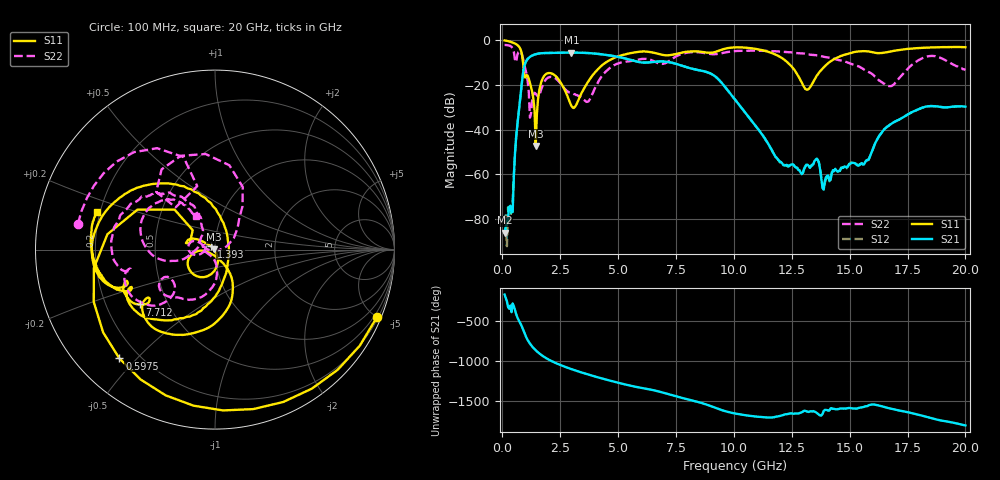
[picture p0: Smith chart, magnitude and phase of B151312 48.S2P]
!  2-Port S-parameters saved by WinCal
! VAR MeasName=S-Parameters (CALIBRATED_DATA) read from VNA (N5244A)
! VAR MeasDate=12/8/2015 5:47:35 PM
! VAR NAME=B151312 48
! VAR FILENAME=B151312 48.S2P
! VAR DATE=12/8/2015 5:47:35 PM
! VAR PHYS_PORTS=1,2
# Hz S DB R 50
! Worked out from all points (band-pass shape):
!   401 points, 100 MHz to 20 GHz, reference 50 ohm
!   highest |S21| = -5.62 dB at 2.986 GHz (marker M1); lowest = -86.1 dB at 100 MHz (marker M2)
!   |S21| within 3 dB of the highest: 1.086 GHz to 5.449 GHz (4.364 GHz wide, 134 % of centre)
!   lowest |S11| = -47.4 dB at 1.443 GHz (marker M3), VSWR 1.01, Z = 49.6 + j0.101 ohm
!   |S11| at or under -10 dB: 896.1 MHz to 4.474 GHz (3.578 GHz wide, 133 % of centre); 12.32 GHz to 14.12 GHz (1.798 GHz wide, 13.6 % of centre)
!   |S22| runs from -34.7 to -2.2 dB; largest |S21 - S12| = 0.0018
!   S11 on the Smith chart (normalised r, x): 100 MHz: 0.29, -4.99; 597.5 MHz: 0.13, -0.45; 1.393 GHz: 0.96, +0.03; 7.712 GHz: 0.35, -0.29; 20 GHz: 0.19, +0.15
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1e8  -0.20 -22.6  -86.13 -169.8  -81.85 -179.3  -2.19 169.3
3.985e8  -0.94 -87.2  -76.92 -30.0  -74.79 8.1  -3.03 129.7
5.975e8  -1.86 -131.3  -43.45 -52.8  -43.50 -52.8  -9.86 132.9
9.4575e8  -15.67 138.9  -11.90 74.9  -11.90 74.8  -10.89 57.6
1.1945e9  -19.11 149.2  -7.51 -63.9  -7.51 -63.9  -34.69 -15.0
1.3935e9  -31.37 139.9  -6.50 -133.2  -6.51 -133.1  -23.60 158.5
1.44325e9  -47.37 166.3  -6.35 -147.4  -6.34 -147.4  -23.99 156.4
1.692e9  -18.49 -91.7  -5.90 152.7  -5.89 152.6  -21.73 -163.1
1.9905e9  -14.77 -130.6  -5.79 98.4  -5.78 98.4  -16.71 -177.6
2.9855e9  -29.43 -144.0  -5.62 -23.0  -5.62 -23.0  -23.76 177.1
3.43325e9  -23.50 -64.8  -5.70 -65.7  -5.70 -65.6  -25.75 -162.9
4.72675e9  -8.51 -84.3  -7.04 -172.5  -7.02 -172.6  -11.89 -101.8
6.7665e9  -6.26 -144.2  -9.58 56.6  -9.58 56.5  -10.47 -148.8
7.71175e9  -5.73 -143.8  -11.36 -19.6  -11.32 -19.7  -6.39 -139.6
1.005e10  -3.28 -175.8  -26.67 141.8  -26.65 141.5  -4.94 -174.0
1.204e10  -7.86 118.6  -54.51 115.4  -54.99 114.6  -5.23 157.2
1.338325e10  -19.56 -47.9  -55.67 167.1  -56.11 169.4  -6.66 138.1
1.388075e10  -12.20 -87.4  -66.76 173.6  -66.85 175.9  -7.49 132.8
1.55225e10  -4.99 -144.7  -54.98 -142.2  -55.09 -142.8  -12.52 116.5
1.67165e10  -5.25 -154.9  -38.06 -152.9  -38.00 -153.6  -20.62 159.4
1.835825e10  -3.42 -174.9  -29.63 96.4  -29.62 95.9  -7.36 165.7
2e10  -3.22 162.3  -29.79 -7.7  -29.89 -8.0  -13.41 119.5
